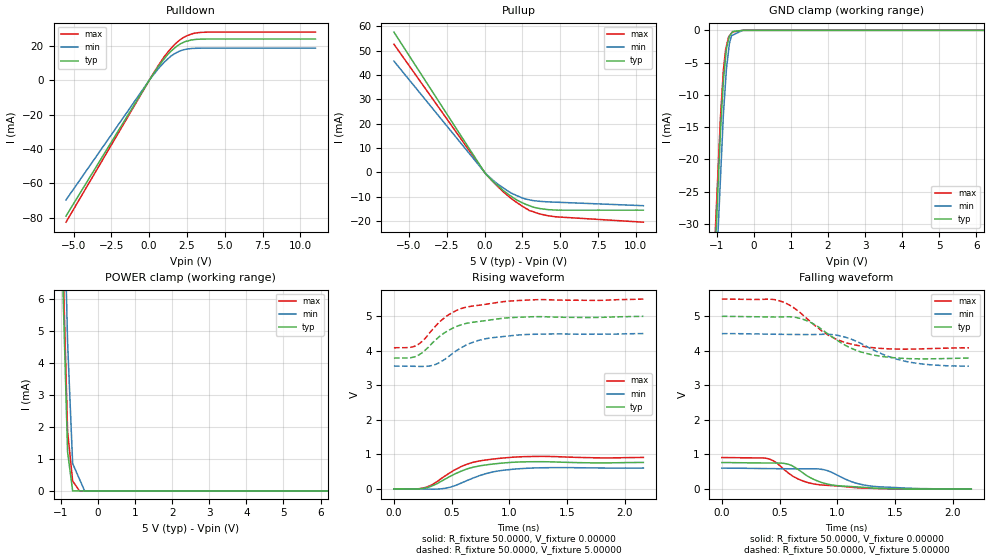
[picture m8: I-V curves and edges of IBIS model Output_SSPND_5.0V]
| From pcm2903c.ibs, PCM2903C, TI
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[Model] Output_SSPND_5.0V
Model_type Output
Vref  = 0.00000V
Cref  = 1.00000pF
Vmeas = 1.65000V
C_comp  2.00000pF 2.00000pF 2.00000pF
| variable   typ   min   max
[Voltage Range]   5.00000V  4.50000V  5.50000V
[POWER Clamp Reference]  5.00000V  4.50000V  5.50000V
[Pullup Reference]   5.00000V  4.50000V  5.50000V
[Pulldown Reference]   0.00000V  0.00000V  0.00000V
[GND Clamp Reference]   0.00000V  0.00000V  0.00000V
[Temperature Range]   25   85   -25
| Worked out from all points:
|   slope of the pulldown table from 0 to 0.75 V, typ, clamps not added: 76.6 ohm
|   slope of the pullup table from 0 to 0.75 V, typ, clamps not added: 156 ohm
|   GND clamp passes 1 mA (typ) near -0.66 V on its own axis
|   POWER clamp passes 1 mA (typ) near -0.80 V on its own axis
|   rising waveform, R_fixture 50.0000, V_fixture 0.00000: 20-80 % time 296ps typ, 298ps min, 286ps max; typ from 0 V to 0.767 V
|   falling waveform, R_fixture 50.0000, V_fixture 0.00000: 20-80 % time 263ps typ, 275ps min, 265ps max; typ from 0.767 V to 0 V
|   falling waveform, R_fixture 50.0000, V_fixture 5.00000: 20-80 % time 347ps typ, 388ps min, 335ps max; typ from 5 V to 3.79 V
|   rising waveform, R_fixture 50.0000, V_fixture 5.00000: 20-80 % time 312ps typ, 307ps min, 303ps max; typ from 3.79 V to 5 V
[GND Clamp]
-5.5V     -619.2mA   -603.6mA   -595.2mA
-4.5V     -488mA     -477.3mA   -468.7mA
-901.3mV  -15.82mA   -23.09mA   -13.56mA
-820.9mV  -7.773mA   -12.94mA   -6.148mA
-760.2mV  -4.088mA   -7.744mA   -2.928mA
-739.9mV  -2.859mA   -6.01mA    -2.442mA
-679.3mV  -1.371mA   -3.023mA   -988.7uA
-659mV    -871.7uA   -2.02mA    -836.6uA
-603mV    -462uA     -835.4uA   -418uA
-562.2mV  -163.1uA   -722.2uA   -247.8uA
-301.5mV  -11.85uA   0A         -9.256uA
11V       0A         0A         0A
[Pulldown]
-5.5V     -79.09mA   -69.68mA   -82.67mA
21.18mV   336.5uA    313.5uA    292.8uA
603mV     8.073mA    6.88mA     8.658mA
1.219V    15.06mA    12.47mA    16.38mA
1.639V    18.6mA     15.42mA    20.6mA
2.08V     21.42mA    17.35mA    23.99mA
2.478V    22.98mA    18.27mA    26.02mA
2.842V    23.7mA     18.7mA     27.25mA
3.52V     24.16mA    18.87mA    28.14mA
11V       24.2mA     18.89mA    28.24mA
[Pullup]
-6V       57.68mA    45.74mA    52.7mA
59.7mV    -625.2uA   -454.7uA   -538.3uA
721.6mV   -4.716mA   -4.145mA   -4.967mA
1.717V    -9.745mA   -8.383mA   -10.59mA
2.218V    -11.72mA   -9.853mA   -12.85mA
2.941V    -13.7mA    -11.31mA   -15.73mA
3.639V    -14.92mA   -11.95mA   -17.12mA
4.179V    -15.37mA   -12.18mA   -17.87mA
4.789V    -15.6mA    -12.33mA   -18.36mA
10.5V     -15.6mA    -13.75mA   -20.54mA
[POWER Clamp]
-6V       212.4mA    254mA      221.1mA
-1.157V   14.91mA    20.8mA     16.08mA
-821mV    1.218mA    4.648mA    1.861mA
-684.2mV  0A         853.7uA    309.4uA
-500mV    0A         368.1uA    0A
-360.4mV  0A         0A         0A
10.5V     0A         0A         0A
[Rising Waveform]
R_fixture = 50.0000
V_fixture = 0.00000
V_fixture_min = 0.00000
V_fixture_max = 0.00000
0s        0V         0V         0V
200ps     -2.106mV   -1.519mV   789.1uV
280ps     31.35mV    -5.11mV    49.24mV
440ps     277.5mV    15.61mV    370.4mV
580ps     510.9mV    165.6mV    644.5mV
680ps     622.5mV    306mV      765.2mV
800ps     696.2mV    445.2mV    840.2mV
940ps     747.9mV    537.4mV    893.2mV
1.2ns     786.6mV    604.7mV    938.9mV
2.16ns    767.1mV    604.4mV    911.4mV
[Falling Waveform]
R_fixture = 50.0000
V_fixture = 0.00000
V_fixture_min = 0.00000
V_fixture_max = 0.00000
0s        767.1mV    604.4mV    911.4mV
400ps     752.6mV    591.1mV    877.7mV
460ps     752.1mV    589.2mV    789.8mV
580ps     712.6mV    586.2mV    453mV
700ps     470.9mV    584.9mV    236.5mV
820ps     244.5mV    584.6mV    133.7mV
980ps     105.8mV    436.1mV    92.89mV
1.14ns    66.97mV    193.2mV    45.36mV
1.28ns    34.73mV    90.18mV    21.58mV
2.16ns    0V         0V         0V
[Falling Waveform]
R_fixture = 50.0000
V_fixture = 5.00000
V_fixture_min = 4.50000
V_fixture_max = 5.50000
0s        5V         4.5V       5.5V
420ps     4.981V     4.484V     5.495V
520ps     4.983V     4.479V     5.426V
620ps     4.979V     4.475V     5.256V
760ps     4.84V      4.472V     4.867V
980ps     4.346V     4.462V     4.354V
1.18ns    3.998V     4.256V     4.153V
1.4ns     3.833V     3.893V     4.068V
1.58ns    3.781V     3.705V     4.05V
2.14ns    3.792V     3.558V     4.089V
[Rising Waveform]
R_fixture = 50.0000
V_fixture = 5.00000
V_fixture_min = 4.50000
V_fixture_max = 5.50000
0s        3.792V     3.558V     4.089V
120ps     3.793V     3.555V     4.093V
200ps     3.851V     3.55V      4.162V
260ps     3.987V     3.549V     4.322V
340ps     4.251V     3.584V     4.638V
480ps     4.606V     3.852V     5.058V
640ps     4.803V     4.188V     5.275V
800ps     4.878V     4.354V     5.352V
1.1ns     4.975V     4.464V     5.462V
2.16ns    5V         4.5V       5.5V
[Ramp]
| variable typ   min   max
dV/dt_r   462.196m/326.348p  364.018m/326.268p  546.248m/307.716p
dV/dt_f   726.536m/347.202p  566.150m/388.409p  847.320m/335.384p
R_load  =  50.0000Ohms
